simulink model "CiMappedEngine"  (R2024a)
settings: Solver=VariableStepAuto  StartTime=0.0  StopTime=inf  RelTol=1e-3  EnableMultiTasking=on
model workspace (MAT data in the model file):
  AccPwrTbl : Simulink.Parameter (value not decoded)
  AccSpdBpts : Simulink.Parameter (value not decoded)
  Cps : Simulink.Parameter (value not decoded)
  NCyl : Simulink.Parameter (value not decoded)
  Pstd : Simulink.Parameter (value not decoded)
  Rair : Simulink.Parameter (value not decoded)
  Sinj : Simulink.Parameter (value not decoded)
  TimeCnstECP : Simulink.Parameter (value not decoded)
  TimeCnstEGR : Simulink.Parameter (value not decoded)
  TimeCnstETC : Simulink.Parameter (value not decoded)
  TimeCnstICP : Simulink.Parameter (value not decoded)
  TimeCnstIVL : Simulink.Parameter (value not decoded)
  TimeCnstSWVA : Simulink.Parameter (value not decoded)
  TimeCnstVCR : Simulink.Parameter (value not decoded)
  TimeCnstVGT : Simulink.Parameter (value not decoded)
  TimeCnstVIRL : Simulink.Parameter (value not decoded)
  TimeCnstWGA : Simulink.Parameter (value not decoded)
  Tstd : Simulink.Parameter (value not decoded)
  Vd : Simulink.Parameter (value not decoded)
  f_air : Simulink.Parameter (value not decoded)
  f_air_3d : Simulink.Parameter (value not decoded)
  f_co : Simulink.Parameter (value not decoded)
  f_co2 : Simulink.Parameter (value not decoded)
  f_co2_3d : Simulink.Parameter (value not decoded)
  f_co_3d : Simulink.Parameter (value not decoded)
  f_eff : Simulink.Parameter (value not decoded)
  f_eff_3d : Simulink.Parameter (value not decoded)
  f_fuel : Simulink.Parameter (value not decoded)
  f_fuel_3d : Simulink.Parameter (value not decoded)
  f_hc : Simulink.Parameter (value not decoded)
  f_hc_3d : Simulink.Parameter (value not decoded)
  f_nox : Simulink.Parameter (value not decoded)
  f_nox_3d : Simulink.Parameter (value not decoded)
  f_pm : Simulink.Parameter (value not decoded)
  f_pm_3d : Simulink.Parameter (value not decoded)
  f_tbrake : Simulink.Parameter (value not decoded)
  f_tbrake_3d : Simulink.Parameter (value not decoded)
  f_tbrake_f_bpt : Simulink.Parameter (value not decoded)
  f_tbrake_n_bpt : Simulink.Parameter (value not decoded)
  f_tbrake_t_bpt : Simulink.Parameter (value not decoded)
  f_texh : Simulink.Parameter (value not decoded)
  f_texh_3d : Simulink.Parameter (value not decoded)
symbols that are objects in the model workspace (value not decoded): Sinj, TimeCnstECP, TimeCnstEGR, TimeCnstETC, TimeCnstICP, TimeCnstIVL, TimeCnstSWVA, TimeCnstVCR, TimeCnstVGT, TimeCnstVIRL, TimeCnstWGA
undefined symbols (not defined in the file or in its folder): CO2, EO
libraries: autolibhevctrlrcommon x1, autolibpowerinfoutils x1, autolibsharedmappedengines x1

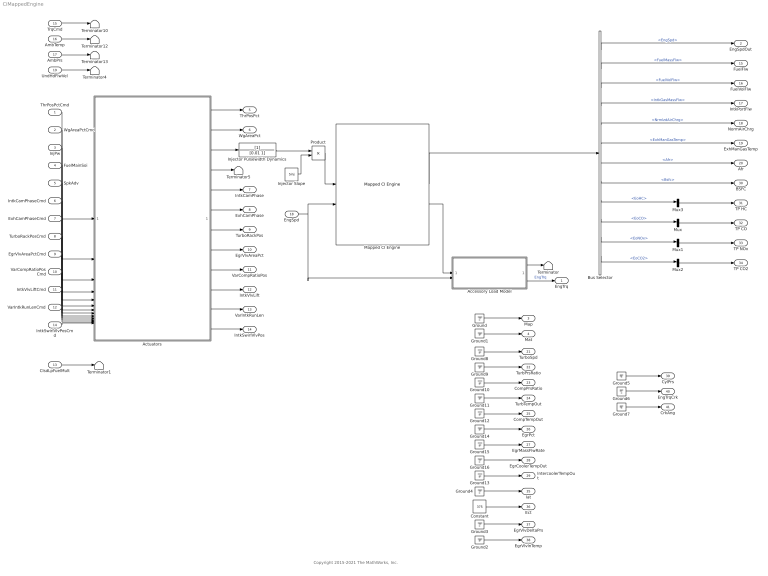
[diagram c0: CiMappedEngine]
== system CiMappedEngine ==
  note: Copyright 2015-2021 The MathWorks, Inc.
  ThrPosPctCmd : Inport
  WgAreaPctCmd : Inport  Port=2
  InjPw : Inport  Port=3
  FuelMainSoi : Inport  Port=4
  SpkAdv : Inport  Port=5
  IntkCamPhaseCmd : Inport  Port=6
  ExhCamPhaseCmd : Inport  Port=7
  TurboRackPosCmd : Inport  Port=8
  EgrVlvAreaPctCmd : Inport  Port=9
  VarCompRatioPosCmd : Inport  Port=10
  IntkVlvLiftCmd : Inport  Port=11
  VarIntkRunLenCmd : Inport  Port=12
  ClsdLpFuelMult : Inport  Port=13  Unit=1
  IntkSwirlVlvPosCmd : Inport  Port=14
  TrqCmd : Inport  Port=15  Unit=N*m
  AmbTemp : Inport  Port=16  Unit=K
  AmbPrs : Inport  Port=17  Unit=Pa
  EngSpd : Inport  Port=18  Interpolate=off
  UndHdFlwVel : Inport  Port=19  Unit=m/s
  Accessory Load Model : Subsystem
  Actuators : Subsystem
  Bus Selector : BusSelector  OutputSignals=EngSpd,FuelMassFlw,FuelVolFlw,IntkGasMassFlw,NrmlzdAirChrg,ExhManGasTemp,Afr,Bsfc,EoHC,EoCO,EoNOx,EoCO2
  Constant : Constant  Value=375
  Ground{,1..16} (17 alike) : Ground
  Injector Pulsewidth Dynamics : TransferFcn  Denominator=[0.01 1]
  Injector Slope : Constant  Value=Sinj
  Mapped CI Engine : autolibsharedmappedengines/Mapped CI Engine  InputCmdPopup=Fuel mass  TurboLagCheckbox=off  EngTmpInpEnbl=off  rowVarName=TrqCmd  f_tbrake_f_bpt=f_tbrake_f_bpt  f_tbrake_t_bpt=f_tbrake_t_bpt  colVarName=EngSpd  f_tbrake_n_bpt=f_tbrake_n_bpt  f_tbrake_engtmp_bpt=[0 1000 1285.71428571429 1571.42857142857 1857.14285714286 2142.85714285714 2428.57142857143 2714.28571428571 3000 3285.71428571429 3571.42857142857 3857.14285714286 4142.85714285714 4428.57142857143 4714.28571428571 5000]  NCyl=NCyl  Cps=Cps  Vd=Vd  Lhv=45e6  Sg=0.832  Rair=Rair  Pstd=Pstd  Tstd=Tstd  Use1=on  Use2=on  Use3=on  Use4=on  Use5=on  Use6=on  Use7=on  Use8=on  Use9=on  Use10=off  f_tbrake_bst=[90, 95, 95, 95, 96, 100, 104, 104, 104, 100, 95, 85, 75, 67, 60, 55]  tau_nat=0.1  tau_bst_rising=1.0  tau_bst_falling=0.7  f_blend_frac=0.01  Name1=Brake Torque  f_tbrake=f_tbrake  f_tbrake_3d=cat(3,[0 -13.1081458684774 -14.1037949635308 -15.5978222223895 -17.1468243988479 -18.57688227287 -19.9284644067992 -21.2542794863055 -22.5937120686825 -24.0017516696912 -25.5203729932636 -27.1667334739623 -28.9776139270543 -31.0652059053262 -33.6382508909905 -36.9873078874202;4.32139921766168 4.32139921766168 4.01696946242645 3.01657627710533 1.85358637804622 0.731516929734549 -0.4275387192502 -1.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  Name2=Air Mass Flow  f_air=f_air  f_air_3d=cat(3,[0 0.00309706924950592 0.00452015548895638 0.00626693492213078 0.00879912183278348 0.0118780141352622 0.0146086872326241 0.0164283363560914 0.017430833463342 0.0179780359688698 0.0183296451622608 0.0185647242912905 0.0186520238218037 0.0185206414129648 0.0181086367688216 0.0174012027671944;0 0.00602292528585861 0.00770048695740641 0.00909327842187188 0.0120300250825315 0.0165547686351833 0.0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  Name3=Fuel Flow  f_fuel=f_fuel  f_fuel_3d=cat(3,[0 0 0 0 0 0 1.96872590895162e-08 1.11497559089192e-07 2.08845127798106e-07 2.82196894845497e-07 3.36789183807035e-07 3.85963069087249e-07 4.43703799512474e-07 5.16303552365966e-07 6.18958920559444e-07 7.66022406381668e-07;0 8.65785362426501e-05 0.00011203764940267 0.000137411179243721 0.00016270746005005 0.000187945932561446 0.00021312794139946 0.0002382669520308 0.000263366151267778 0.0002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  Name4=Exhaust Temperature  f_texh=f_texh  f_texh_3d=cat(3,[358.711368346279 358.711368346279 367.983969839492 375.766236578521 379.824873013623 380.377581918888 381.168020674094 384.445628826361 389.975238414473 397.276334747317 406.687273458426 418.723655106797 433.343123892387 449.95713948592 467.887943023565 486.766068837338;410.521929895625 410.521929895625 418.333326741241 425.972726120476 430.142630320378 430.676036782825 433.565609920626 439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  Name5=[300 300 300 300 300 300 300 300 300 300 300 300 300 300 300 300 300 300 300 300;297.183191911082 296.381813482439 298.389346568793 300 300 300 300 300 300 300 300 300 294.67266237158 289.737568904754 289.12856875624 291.461389167304 295.189395927038 297.348559050166 294.666946050542 286.881979097439;300 300 300 300 300 300 300 300 300 300 300 295.311694583484 288.854995920935 285.748220888279 286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  f_eff=f_eff  f_eff_3d=cat(3,[0 300 300 300 300 300 300 300 300 300 300 300 300 300 300 300;0 297.183191911082 296.426611034351 298.164901875909 299.729890418369 300 300 300 300 300 300 300 300 298.246280159588 293.323941175677 289.605177568121;0 300 300 300 300 300 300 300 300 300 300 300 298.194565616 293.186197508235 288.005939390271 285.831249666291;0 300 300 300 300 298.830780543781 288.45010517615 269.198351279529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  Name6=EO HC  f_hc=f_hc  f_hc_3d=cat(3,[0 5.41090940906478e-10 5.82277246149883e-10 6.06293368838046e-10 5.93131722841061e-10 5.23839609255542e-10 3.91944606807851e-10 2.09234652579032e-10 5.4438838779207e-11 0 0 0 0 0 0 8.76094213556711e-14;0 9.66157682132999e-10 1.14171380367877e-09 1.3085398373022e-09 1.436731750244e-09 1.50140710830807e-09 1.49054993471198e-09 1.4037387429616e-09 1.25592949365723e-09 1.08480750810599e-09 9.48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  Name7=EO CO  f_co=f_co  f_co_3d=cat(3,[0 1.67160387663193e-08 1.20397081499173e-08 9.52610812306698e-09 8.36631447493353e-09 7.72547679934784e-09 6.8319182072918e-09 5.0682750909637e-09 2.053636244448e-09 2.64830540952401e-10 0 0 0 0 0 0;0 1.8291738663811e-08 1.5484401198941e-08 1.54411575714574e-08 1.72039510086271e-08 1.97426073770272e-08 2.2067112907845e-08 2.33532431661193e-08 2.30715889811663e-08 2.1102272015203e-08 1.78032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  Name8=EO NOx  f_nox=f_nox  f_nox_3d=cat(3,[0 3.21218888850422e-07 1.79563354015778e-08 0 0 0 0 7.27128716806088e-09 2.382216838202e-07 4.44107113496821e-07 4.91577691057171e-07 5.14872133427744e-07 5.86973145400533e-07 7.14855423266785e-07 9.07945412418829e-07 1.1362893758644e-06;0 0 0 0 0 4.01712899078589e-07 9.14038671754761e-07 1.21206139039062e-06 1.258219700583e-06 1.15680571609299e-06 9.88518749662651e-07 7.9819948867334e-07 6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  Name9=EO CO2  f_co2=f_co2  f_co2_3d=cat(3,[0 0 0 0 0 0 0 0 0 0 0 0 0 0 0 0;0 0 0.00030365633115907 0.000477004645283182 0.000566806090053379 0.000616848625254133 0.000657878888237009 0.000704613499127597 0.000759308138241543 0.000818372753847269 0.000877510431637555 0.00093411034677875 0.000987559137783125 0.00103750226880644 0.00108100059676674 0.00111208043085771;0 0.000531197372565358 0.000833769373636657 0.00101208952923391 0.00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  Name10=Brake Torque  f_pm=f_pm  f_pm_3d=cat(3,[0 0 0 0 0 0 0 0 0 0 0 0 0 0 0 0;0 0 0 0 0 0 0 0 0 0 0 0 0 0 0 0;0 0 0 0 0 0 0 0 0 0 0 0 0 0 0 0;0 0 0 0 0 0 0 0 0 0 0 0 0 0 0 0;0 0 0 0 0 0 0 0 0 0 0 0 0 0 0 0;0 0 0 0 0 0 0 0 0 0 0 0 0 0 0 0;0 0 0 0 0 0 0 0 0 0 0 0 0 0 0 0;0 0 0 0 0 0 0 0 0 0 0 0 0 0 0 0;0 0 0 0 0 0 0 0 0 0 0 0 0 0 0 0;0 0 0 0 0 0 0 0 0 0 0 0 0 0 0 0;0 0 0 0 0 0 0 0 0 0 0 0 0 0 0 0;0 0 0 0 0 0 0 0 0 0 0 0 0 0 0 0;0 0 0 0 0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  aMode=1  CalMapsFuelCmdData={'', '', 'MappedEngine-Torque', 'MappedEngine-Nonfiring'}  CalMapsTrqCmdData={'', '', 'MappedEngine-Torque', 'MappedEngine-Nonfiring'}
  Mux{,1..3} (4 alike) : Mux  Inputs=1
  Product : Product
  Terminator{,1,4..5,10,12..13} (7 alike) : Terminator
  EngTrq : Outport  Unit=N*m  VectorParamsAs1DForOutWhenUnconnected=off
  EngSpdOut : Outport  Port=2  VectorParamsAs1DForOutWhenUnconnected=off
  Map : Outport  Port=3  Unit=Pa  VectorParamsAs1DForOutWhenUnconnected=off
  Mat : Outport  Port=4  Unit=K  VectorParamsAs1DForOutWhenUnconnected=off
  ThrPosPct : Outport  Port=5  VectorParamsAs1DForOutWhenUnconnected=off
  WgAreaPct : Outport  Port=6  VectorParamsAs1DForOutWhenUnconnected=off
  IntkCamPhase : Outport  Port=7  VectorParamsAs1DForOutWhenUnconnected=off
  ExhCamPhase : Outport  Port=8  VectorParamsAs1DForOutWhenUnconnected=off
  TurboRackPos : Outport  Port=9  VectorParamsAs1DForOutWhenUnconnected=off
  EgrVlvAreaPct : Outport  Port=10  VectorParamsAs1DForOutWhenUnconnected=off
  VarCompRatioPos : Outport  Port=11  VectorParamsAs1DForOutWhenUnconnected=off
  IntkVlvLift : Outport  Port=12  VectorParamsAs1DForOutWhenUnconnected=off
  VarIntkRunLen : Outport  Port=13  VectorParamsAs1DForOutWhenUnconnected=off
  IntkSwirlVlvPos : Outport  Port=14  VectorParamsAs1DForOutWhenUnconnected=off
  FuelFlw : Outport  Port=15  VectorParamsAs1DForOutWhenUnconnected=off
  FuelVolFlw : Outport  Port=16  VectorParamsAs1DForOutWhenUnconnected=off
  IntkPortFlw : Outport  Port=17  VectorParamsAs1DForOutWhenUnconnected=off
  NormAirChrg : Outport  Port=18  VectorParamsAs1DForOutWhenUnconnected=off
  ExhManGasTemp : Outport  Port=19  VectorParamsAs1DForOutWhenUnconnected=off
  Afr : Outport  Port=20  Unit=1  VectorParamsAs1DForOutWhenUnconnected=off
  TurboSpd : Outport  Port=21  Unit=rad/s  VectorParamsAs1DForOutWhenUnconnected=off
  TurbPrsRatio : Outport  Port=22  Unit=1  VectorParamsAs1DForOutWhenUnconnected=off
  CompPrsRatio : Outport  Port=23  Unit=1  VectorParamsAs1DForOutWhenUnconnected=off
  TurbTempOut : Outport  Port=24  Unit=K  VectorParamsAs1DForOutWhenUnconnected=off
  CompTempOut : Outport  Port=25  Unit=K  VectorParamsAs1DForOutWhenUnconnected=off
  EgrPct : Outport  Port=26  Unit=%  VectorParamsAs1DForOutWhenUnconnected=off
  EgrMassFlwRate : Outport  Port=27  Unit=kg/s  VectorParamsAs1DForOutWhenUnconnected=off
  EgrCoolerTempOut : Outport  Port=28  Unit=K  VectorParamsAs1DForOutWhenUnconnected=off
  IntercoolerTempOut : Outport  Port=29  Unit=K  VectorParamsAs1DForOutWhenUnconnected=off
  BSFC : Outport  Port=30  VectorParamsAs1DForOutWhenUnconnected=off
  TP HC : Outport  Port=31  VectorParamsAs1DForOutWhenUnconnected=off
  TP CO : Outport  Port=32  VectorParamsAs1DForOutWhenUnconnected=off
  TP NOx : Outport  Port=33  VectorParamsAs1DForOutWhenUnconnected=off
  TP CO2 : Outport  Port=34  VectorParamsAs1DForOutWhenUnconnected=off
  Iat : Outport  Port=35  Unit=K  VectorParamsAs1DForOutWhenUnconnected=off
  Ect : Outport  Port=36  Unit=K  VectorParamsAs1DForOutWhenUnconnected=off
  EgrVlvDeltaPrs : Outport  Port=37  Unit=Pa  VectorParamsAs1DForOutWhenUnconnected=off
  EgrVlvInTemp : Outport  Port=38  Unit=K  VectorParamsAs1DForOutWhenUnconnected=off
  CylPrs : Outport  Port=39  VectorParamsAs1DForOutWhenUnconnected=off
  EngTrqCrk : Outport  Port=40  VectorParamsAs1DForOutWhenUnconnected=off
  CrkAng : Outport  Port=41  VectorParamsAs1DForOutWhenUnconnected=off
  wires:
  InjPw/1 -> Actuators/3(InjPwCmd)
  EngSpd/1 -> Accessory Load Model/2(EngSpd), Mapped CI Engine/2
  Accessory Load Model/2(EngTrqOut) -> EngTrq/1  "EngTrq"
  Product/1 -> Mapped CI Engine/1
  Injector Slope/1 -> Product/2
  AmbTemp/1 -> Terminator12/1
  Mapped CI Engine/1 -> Bus Selector/1
  Ground/1 -> Map/1
  Ground1/1 -> Mat/1
  TrqCmd/1 -> Terminator10/1
  AmbPrs/1 -> Terminator13/1
  UndHdFlwVel/1 -> Terminator4/1
  Bus Selector/6 -> ExhManGasTemp/1  "<ExhManGasTemp>"
  Bus Selector/7 -> Afr/1  "<Afr>"
  Bus Selector/1 -> EngSpdOut/1  "<EngSpd>"
  Bus Selector/2 -> FuelFlw/1  "<FuelMassFlw>"
  Bus Selector/4 -> IntkPortFlw/1  "<IntkGasMassFlw>"
  Bus Selector/9 -> Mux3/1  "<EoHC>"
  Bus Selector/10 -> Mux/1  "<EoCO>"
  Bus Selector/11 -> Mux1/1  "<EoNOx>"
  Bus Selector/12 -> Mux2/1  "<EoCO2>"
  Mux3/1 -> TP HC/1
  Mux/1 -> TP CO/1
  Mux1/1 -> TP NOx/1
  Mux2/1 -> TP CO2/1
  Bus Selector/8 -> BSFC/1  "<Bsfc>"
  Bus Selector/5 -> NormAirChrg/1  "<NrmlzdAirChrg>"
  Ground8/1 -> TurboSpd/1
  Ground9/1 -> TurbPrsRatio/1
  Ground10/1 -> CompPrsRatio/1
  Ground11/1 -> TurbTempOut/1
  Ground12/1 -> CompTempOut/1
  Ground13/1 -> IntercoolerTempOut/1
  Ground14/1 -> EgrPct/1
  Ground15/1 -> EgrMassFlwRate/1
  Ground16/1 -> EgrCoolerTempOut/1
  Injector Pulsewidth Dynamics/1 -> Product/1
  ThrPosPctCmd/1 -> Actuators/1(ThrPosPctCmd)
  WgAreaPctCmd/1 -> Actuators/2(WgAreaPctCmd)
  Actuators/3(InjPw) -> Injector Pulsewidth Dynamics/1
  Actuators/1(ThrPosPct) -> ThrPosPct/1
  Actuators/2(WgAreaPct) -> WgAreaPct/1
  Actuators/4(FuelMainSoi) -> Terminator5/1
  FuelMainSoi/1 -> Actuators/4(FuelMainSoiCmd)
  SpkAdv/1 -> Actuators/5(SpkAdvCmd)
  IntkCamPhaseCmd/1 -> Actuators/6(IntkCamPhaseCmd)
  ExhCamPhaseCmd/1 -> Actuators/7(ExhCamPhaseCmd)
  TurboRackPosCmd/1 -> Actuators/8(TurboRackPosCmd)
  EgrVlvAreaPctCmd/1 -> Actuators/9(EgrVlvAreaPctCmd)
  VarCompRatioPosCmd/1 -> Actuators/10(VarCompRatioPosCmd)
  IntkVlvLiftCmd/1 -> Actuators/11(IntkVlvLiftCmd)
  VarIntkRunLenCmd/1 -> Actuators/12(VarIntkRunLenCmd)
  ClsdLpFuelMult/1 -> Terminator1/1
  IntkSwirlVlvPosCmd/1 -> Actuators/13(IntkSwirlVlvPosCmd)
  Actuators/12(IntkSwirlVlvPos) -> IntkSwirlVlvPos/1
  Actuators/10(IntkVlvLift) -> IntkVlvLift/1
  Actuators/9(VarCompRatioPos) -> VarCompRatioPos/1
  Actuators/8(EgrVlvAreaPct) -> EgrVlvAreaPct/1
  Actuators/7(TurboRackPos) -> TurboRackPos/1
  Actuators/6(ExhCamPhase) -> ExhCamPhase/1
  Actuators/5(IntkCamPhase) -> IntkCamPhase/1
  Actuators/11(VarIntkRunLen) -> VarIntkRunLen/1
  Constant/1 -> Ect/1
  Ground3/1 -> EgrVlvDeltaPrs/1
  Ground2/1 -> EgrVlvInTemp/1
  Ground4/1 -> Iat/1
  Mapped CI Engine/2 -> Accessory Load Model/1(EngTrqIn)
  Accessory Load Model/1(PwrInfo) -> Terminator/1
  Bus Selector/3 -> FuelVolFlw/1  "<FuelVolFlw>"
  Ground5/1 -> CylPrs/1
  Ground6/1 -> EngTrqCrk/1
  Ground7/1 -> CrkAng/1

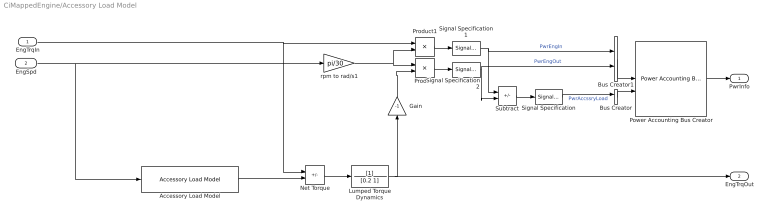
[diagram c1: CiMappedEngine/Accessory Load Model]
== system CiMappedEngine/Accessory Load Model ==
  EngTrqIn : Inport
  EngSpd : Inport  Port=2
  Accessory Load Model : autolibhevctrlrcommon/Accessory Load Model  AccPwrTbl=AccPwrTbl  AccSpdBpts=AccSpdBpts
  Bus Creator : BusCreator  Inputs=1
  Bus Creator1 : BusCreator  Inputs=2
  Gain : Gain  Gain=-1
  Lumped Torque Dynamics : TransferFcn  Denominator=[0.2 1]
  Net Torque : Sum  Inputs=+-
  Power Accounting Bus Creator : autolibpowerinfoutils/Power Accounting Bus Creator  AssctBlkSelPopup=Parent  RefBlkName='libraryname/blkname'  PwrTrnsfrdCheckBox=on  PwrNotTrnsfrdCheckBox=on  PwrStoredCheckBox=off  aMode=aMode
  Product : Product
  Product1 : Product
  Signal Specification : SignalSpecification  Unit=W
  Signal Specification1 : SignalSpecification  Unit=W
  Signal Specification2 : SignalSpecification  Unit=W
  Subtract : Sum  Inputs=--
  rpm to rad/s1 : Gain  Gain=pi/30
  PwrInfo : Outport  VectorParamsAs1DForOutWhenUnconnected=off
  EngTrqOut : Outport  Port=2  Unit=N*m  VectorParamsAs1DForOutWhenUnconnected=off
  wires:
  Accessory Load Model/1 -> Net Torque/2
  EngSpd/1 -> Accessory Load Model/1, rpm to rad/s1/1
  Lumped Torque Dynamics/1 -> EngTrqOut/1, Gain/1
  Net Torque/1 -> Lumped Torque Dynamics/1
  Bus Creator/1 -> Power Accounting Bus Creator/2
  Bus Creator1/1 -> Power Accounting Bus Creator/1
  EngTrqIn/1 -> Product1/1, Net Torque/1
  Subtract/1 -> Signal Specification/1
  Signal Specification/1 -> Bus Creator/1  "PwrAccssryLoad"
  Power Accounting Bus Creator/1 -> PwrInfo/1
  Product/1 -> Signal Specification2/1
  Product1/1 -> Signal Specification1/1
  rpm to rad/s1/1 -> Product1/2, Product/1
  Signal Specification1/1 -> Subtract/1, Bus Creator1/1  "PwrEngIn"
  Signal Specification2/1 -> Subtract/2, Bus Creator1/2  "PwrEngOut"
  Gain/1 -> Product/2

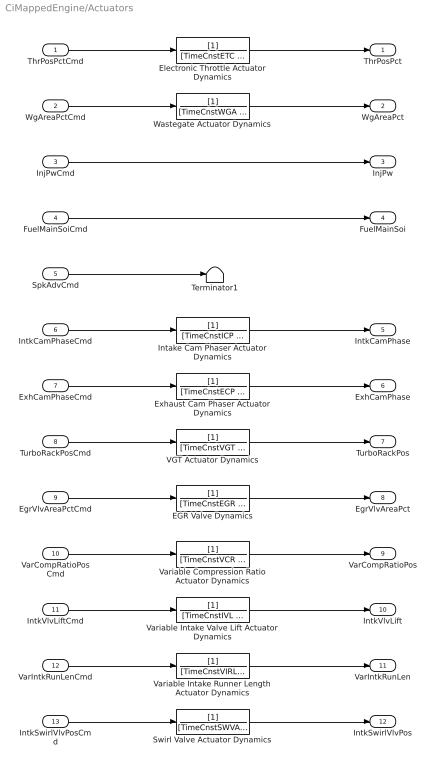
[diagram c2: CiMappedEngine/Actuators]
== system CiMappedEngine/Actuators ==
  ThrPosPctCmd : Inport  Unit=%
  WgAreaPctCmd : Inport  Port=2  Unit=%
  InjPwCmd : Inport  Port=3  Unit=ms
  FuelMainSoiCmd : Inport  Port=4  Unit=deg
  SpkAdvCmd : Inport  Port=5  Unit=deg
  IntkCamPhaseCmd : Inport  Port=6  Unit=deg
  ExhCamPhaseCmd : Inport  Port=7  Unit=deg
  TurboRackPosCmd : Inport  Port=8  Unit=1
  EgrVlvAreaPctCmd : Inport  Port=9  Unit=%
  VarCompRatioPosCmd : Inport  Port=10
  IntkVlvLiftCmd : Inport  Port=11
  VarIntkRunLenCmd : Inport  Port=12
  IntkSwirlVlvPosCmd : Inport  Port=13
  EGR Valve Dynamics : TransferFcn  Denominator=[TimeCnstEGR 1]
  Electronic Throttle Actuator Dynamics : TransferFcn  Denominator=[TimeCnstETC 1]
  Exhaust Cam Phaser Actuator Dynamics : TransferFcn  Denominator=[TimeCnstECP 1]
  Intake Cam Phaser Actuator Dynamics : TransferFcn  Denominator=[TimeCnstICP 1]
  Swirl Valve Actuator Dynamics : TransferFcn  Denominator=[TimeCnstSWVA 1]
  Terminator1 : Terminator
  VGT Actuator Dynamics : TransferFcn  Denominator=[TimeCnstVGT 1]
  Variable Compression Ratio Actuator Dynamics : TransferFcn  Denominator=[TimeCnstVCR 1]
  Variable Intake Runner Length Actuator Dynamics : TransferFcn  Denominator=[TimeCnstVIRL 1]
  Variable Intake Valve Lift Actuator Dynamics : TransferFcn  Denominator=[TimeCnstIVL 1]
  Wastegate Actuator Dynamics : TransferFcn  Denominator=[TimeCnstWGA 1]
  ThrPosPct : Outport  Unit=%  VectorParamsAs1DForOutWhenUnconnected=off
  WgAreaPct : Outport  Port=2  Unit=%  VectorParamsAs1DForOutWhenUnconnected=off
  InjPw : Outport  Port=3  VectorParamsAs1DForOutWhenUnconnected=off
  FuelMainSoi : Outport  Port=4  VectorParamsAs1DForOutWhenUnconnected=off
  IntkCamPhase : Outport  Port=5  Unit=deg  VectorParamsAs1DForOutWhenUnconnected=off
  ExhCamPhase : Outport  Port=6  Unit=deg  VectorParamsAs1DForOutWhenUnconnected=off
  TurboRackPos : Outport  Port=7  Unit=1  VectorParamsAs1DForOutWhenUnconnected=off
  EgrVlvAreaPct : Outport  Port=8  Unit=%  VectorParamsAs1DForOutWhenUnconnected=off
  VarCompRatioPos : Outport  Port=9  VectorParamsAs1DForOutWhenUnconnected=off
  IntkVlvLift : Outport  Port=10  VectorParamsAs1DForOutWhenUnconnected=off
  VarIntkRunLen : Outport  Port=11  VectorParamsAs1DForOutWhenUnconnected=off
  IntkSwirlVlvPos : Outport  Port=12  VectorParamsAs1DForOutWhenUnconnected=off
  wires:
  SpkAdvCmd/1 -> Terminator1/1
  EgrVlvAreaPctCmd/1 -> EGR Valve Dynamics/1
  TurboRackPosCmd/1 -> VGT Actuator Dynamics/1
  EGR Valve Dynamics/1 -> EgrVlvAreaPct/1
  VGT Actuator Dynamics/1 -> TurboRackPos/1
  InjPwCmd/1 -> InjPw/1
  VarIntkRunLenCmd/1 -> Variable Intake Runner Length Actuator Dynamics/1
  VarCompRatioPosCmd/1 -> Variable Compression Ratio Actuator Dynamics/1
  IntkCamPhaseCmd/1 -> Intake Cam Phaser Actuator Dynamics/1
  ExhCamPhaseCmd/1 -> Exhaust Cam Phaser Actuator Dynamics/1
  ThrPosPctCmd/1 -> Electronic Throttle Actuator Dynamics/1
  WgAreaPctCmd/1 -> Wastegate Actuator Dynamics/1
  IntkSwirlVlvPosCmd/1 -> Swirl Valve Actuator Dynamics/1
  IntkVlvLiftCmd/1 -> Variable Intake Valve Lift Actuator Dynamics/1
  FuelMainSoiCmd/1 -> FuelMainSoi/1
  Electronic Throttle Actuator Dynamics/1 -> ThrPosPct/1
  Wastegate Actuator Dynamics/1 -> WgAreaPct/1
  Exhaust Cam Phaser Actuator Dynamics/1 -> ExhCamPhase/1
  Intake Cam Phaser Actuator Dynamics/1 -> IntkCamPhase/1
  Swirl Valve Actuator Dynamics/1 -> IntkSwirlVlvPos/1
  Variable Intake Runner Length Actuator Dynamics/1 -> VarIntkRunLen/1
  Variable Intake Valve Lift Actuator Dynamics/1 -> IntkVlvLift/1
  Variable Compression Ratio Actuator Dynamics/1 -> VarCompRatioPos/1
